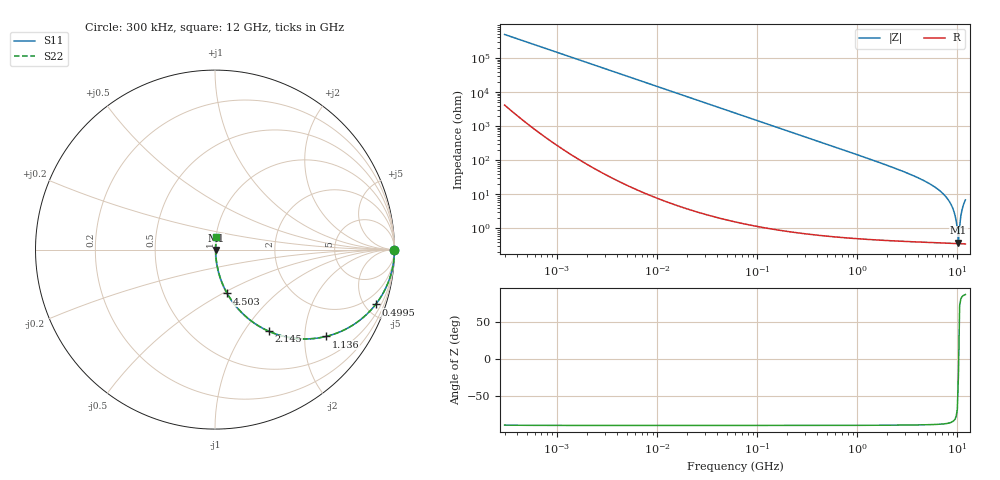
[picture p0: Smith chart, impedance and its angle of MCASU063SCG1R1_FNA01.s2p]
! MCASU063SCG1R1_FNA01  S-PARAMETER MODEL  ( Standard Model )
! Model Generated by TAIYO YUDEN Corporation (http://www.ty-top.com)
! Version 1.0
! TAIYO YUDEN Control No. 230609
! Copyright(c) 2023 TAIYO YUDEN CO.,LTD. All Rights Reserved.
! Product Description (link to TY-COMPAS)
! https://ds.yuden.co.jp/TYCOMPAS/or/detail?pn=MCASU063SCG1R1BFNA01&u=M
! Products Name : Multilayer Ceramic Capacitors
! Characteristics :
!  Capacitance : 1.1 [pF] , Rated Voltage : 50 [V] , TCC : CG / C0G
!  Case Size : 0.6 x 0.3 / 0.024 x 0.012 [mm/inch] , Thickness : 0.3 / 0.012 [mm/inch]
!  (Conditions: Temperature = 25 [degC] , DC Bias Voltage = 0 [V])
! External Node Assignments :
!  1  o---| |---o  2
! GND o---------o GND
! Frequency Range : 0.3MHz  -  12000MHz  [ 401 STEP ]
# MHZ S RI R 50
! Freq[MHz].  S11 Real  S11 Imag  S21 Real  S21 Imag  S12 Real  S12 Imag  S22 Real  S22 Imag
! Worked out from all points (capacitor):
!   401 points, 300 kHz to 12 GHz, reference 50 ohm
!   read as one part in series: C = 1.09 pF near 316.3 kHz
!   lowest |Z| = 383 mohm at 10.24 GHz (marker M1)
!   series resonance near 10.27 GHz, so ESL is about 220 pH
!   S11 on the Smith chart (normalised r, x): 300 kHz: open; 499.5 MHz: 1.01, -5.85; 1.136 GHz: 1.01, -2.55; 2.145 GHz: 1.01, -1.31; 4.503 GHz: 1.01, -0.53; 12 GHz: 1.01, +0.14
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0.3  1 -0.000205  1.78e-06 0.000205  1.78e-06 0.000205  1 -0.000205
1.769972  1 -0.00121  2.83e-06 0.00121  2.83e-06 0.00121  1 -0.00121
10.44266  0.9999 -0.00713  5.45e-05 0.00713  5.45e-05 0.00713  0.9999 -0.00713
60  0.9983 -0.0409  0.0017 0.0409  0.0017 0.0409  0.9983 -0.0409
353.9943  0.9444 -0.2283  0.0556 0.2283  0.0556 0.2283  0.9444 -0.2283
499.5319  0.895 -0.3056  0.105 0.3056  0.105 0.3056  0.895 -0.3056
1135.593  0.6186 -0.4838  0.3814 0.4838  0.3814 0.4838  0.6186 -0.4838
2088.533  0.3127 -0.4603  0.6873 0.4603  0.6873 0.4603  0.3127 -0.4603
2144.601  0.3006 -0.4552  0.6994 0.4552  0.6994 0.4552  0.3006 -0.4552
4502.883  0.068 -0.2443  0.932 0.2443  0.932 0.2443  0.068 -0.2443
6354.153  0.0235 -0.1388  0.9765 0.1388  0.9765 0.1388  0.0235 -0.1388
7854.144  0.00966 -0.0769  0.9903 0.0769  0.9903 0.0769  0.00966 -0.0769
8966.534  0.00517 -0.039  0.9948 0.039  0.9948 0.039  0.00517 -0.039
9454.42  0.0042 -0.024  0.9958 0.024  0.9958 0.024  0.0042 -0.024
9708.23  0.00388 -0.0165  0.9961 0.0165  0.9961 0.0165  0.00388 -0.0165
9968.853  0.00368 -0.00893  0.9963 0.00893  0.9963 0.00893  0.00368 -0.00893
10236.47  0.00359 -0.00131  0.9964 0.00131  0.9964 0.00131  0.00359 -0.00131
10511.28  0.00369 0.0109  0.9963 -0.0109  0.9963 -0.0109  0.00369 0.0109
10793.46  0.00406 0.0223  0.9959 -0.0223  0.9959 -0.0223  0.00406 0.0223
11083.22  0.00469 0.0337  0.9953 -0.0337  0.9953 -0.0337  0.00469 0.0337
11380.75  0.00561 0.0453  0.9944 -0.0453  0.9944 -0.0453  0.00561 0.0453
12000  0.00817 0.068  0.9918 -0.068  0.9918 -0.068  0.00817 0.068
